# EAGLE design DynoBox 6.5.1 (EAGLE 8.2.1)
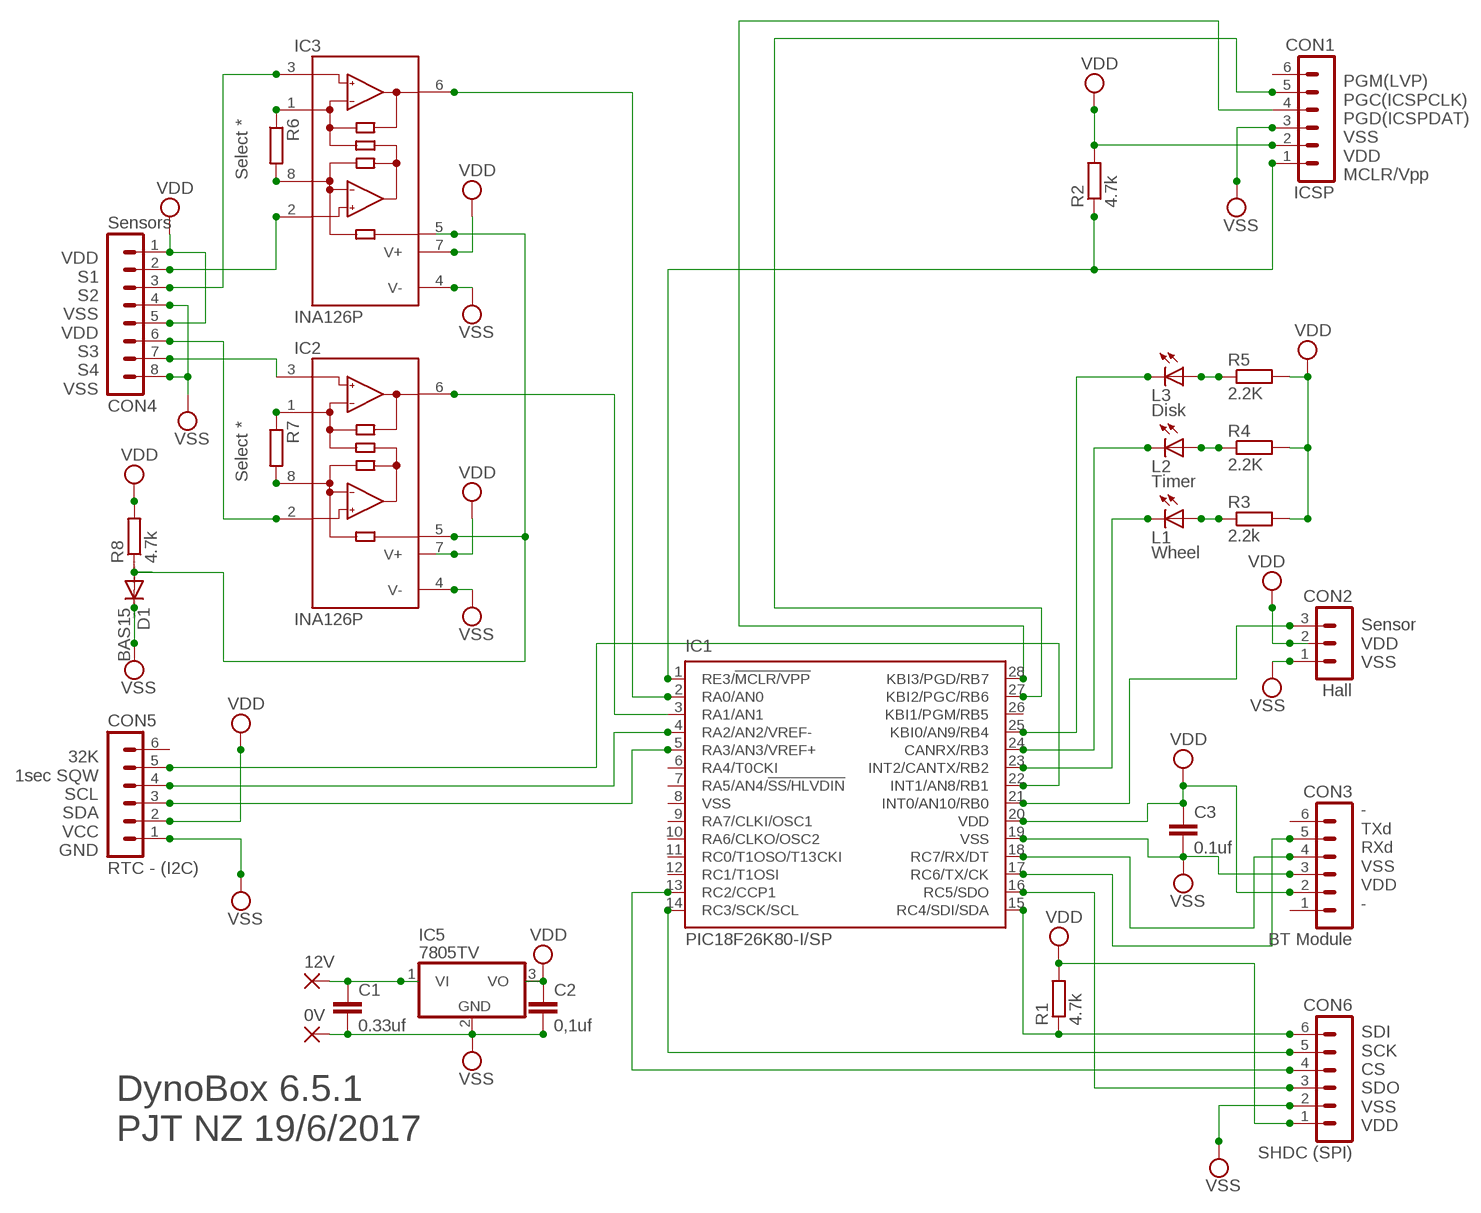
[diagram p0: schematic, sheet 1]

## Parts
0V  1,6/0,9  [1,6/0,9]
12V  1,6/0,9  [1,6/0,9]
C1  0.33uf  C-EU025-040X050  [C025-040X050]
C2  0,1uf  C-EU025-040X050  [C025-040X050]
C3  0.1uf  C-EU025-025X050  [C025-025X050]
CON1  ICSP  MA06-1  [MA06-1]
CON2  Hall  MA03-1  [MA03-1]
CON3  BT Module  MA06-1  [MA06-1]
CON4  Sensors  MA08-1  [MA08-1]
CON5  RTC - (I2C)  MA06-1  [MA06-1]
CON6  SHDC (SPI)  MA06-1  [MA06-1]
D1  BAS15  [DO34-7]
IC1  PIC18F26K80-I/SP  PIC18F2580-I/SP  [DIL28-3]
IC2  INA126P  [DIL08]
IC3  INA126P  [DIL08]
IC5  7805TV  [TO220V]
L1  Wheel  LED3MM  [LED3MM]
L2  Timer  LED3MM  [LED3MM]
L3  Disk  LED3MM  [LED3MM]
R1  4.7k  R-EU_0204/7  [0204/7]
R2  4.7k  R-EU_0204/7  [0204/7]
R3  2.2k  R-EU_0207/2V  [0207/2V]
R4  2.2K  R-EU_0207/2V  [0207/2V]
R5  2.2K  R-EU_0207/2V  [0207/2V]
R6  Select *  R-EU_0204/7  [0204/7]
R7  Select *  R-EU_0204/7  [0204/7]
R8  4.7k  R-EU_0204/7  [0204/7]

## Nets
1SEC: CON5.5 IC1.22(INT1/AN8/RB1)
N$1: IC2.8(RG) R7.2
N$2: IC2.1(RG) R7.1
N$3: L3.A R5.1
N$4: L2.A R4.1
N$6: L1.A R3.1
N$9: D1.A IC2.5(REF) IC3.5(REF) R8.1
N$10: 12V.1(P) C1.1 IC5.1(VI)
N$11: CON1.1 IC1.1(RE3/!MCLR/VPP) R2.1
N$12: CON1.4 IC1.28(KBI3/PGD/RB7)
N$13: CON1.5 IC1.27(KBI2/PGC/RB6)
N$16: CON6.6 IC1.15(RC4/SDI/SDA) R1.1
N$17: IC1.2(RA0/AN0) IC3.6(OUT)
N$18: IC1.3(RA1/AN1) IC2.6(OUT)
N$19: CON3.4 IC1.18(RC7/RX/DT)
N$20: IC3.8(RG) R6.2
N$21: CON3.5 IC1.17(RC6/TX/CK)
N$22: CON6.5 IC1.14(RC3/SCK/SCL)
N$23: IC3.1(RG) R6.1
N$28: CON6.3 IC1.16(RC5/SDO)
N$33: IC1.24(CANRX/RB3) L2.K(C)
N$34: IC1.23(INT2/CANTX/RB2) L1.K(C)
N$36: CON2.3 IC1.21(INT0/AN10/RB0)
N$37: CON5.3 IC1.5(RA3/AN3/VREF+)
N$38: CON5.4 IC1.4(RA2/AN2/VREF-)
N$39: CON6.4 IC1.13(RC2/CCP1)
N$41: IC1.25(KBI0/AN9/RB4) L3.K(C)
S1: CON4.2 IC3.2(-IN)
S2: CON4.3 IC3.3(+IN)
S3: CON4.6 IC2.2(-IN)
S4: CON4.7 IC2.3(+IN)
VDD: C2.1 C3.1 CON1.2 CON2.2 CON3.2 CON4.1 CON4.5 CON5.2 CON6.1 IC1.20(VDD) IC2.7(V+) IC3.7(V+) IC5.3(VO) R1.2 R2.2 R3.2 R4.2 R5.2 R8.2
VSS: 0V.1(P) C1.2 C2.2 C3.2 CON1.3 CON2.1 CON3.3 CON4.4 CON4.8 CON5.1 CON6.2 D1.C IC1.19(VSS) IC2.4(V-) IC3.4(V-) IC5.2(GND)
Unconnected: CON1.6 CON3.1 CON3.6 CON5.6 IC1.6(RA4/T0CKI) IC1.7(RA5/AN4/!SS/HLVDIN) IC1.9(RA7/CLKI/OSC1) IC1.10(RA6/CLKO/OSC2) IC1.11(RC0/T1OSO/T13CKI) IC1.12(RC1/T1OSI) IC1.26(KBI1/PGM/RB5)

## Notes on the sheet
- PGM(LVP)
  PGC(ICSPCLK)
  PGD(ICSPDAT)
  VSS
  VDD
  MCLR/Vpp
- VDD
  S1
  S2
  VSS
  VDD
  S3
  S4
  VSS
- Sensor
  VDD
  VSS
- 32K
  1sec SQW
  SCL
  SDA
  VCC
  GND
- -
  TXd
  RXd
  VSS
  VDD
  -
- SDI
  SCK
  CS
  SDO
  VSS
  VDD
- DynoBox 6.5.1
  PJT NZ 19/6/2017

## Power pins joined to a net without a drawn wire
VSS: IC1.8(VSS)

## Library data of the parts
0V 12V = wirepad:1,6/0,9: THROUGH-HOLE PAD
C1 C2 = rcl:C-EU: CAPACITOR, European symbol
C3 = resistor:C-EU: CAPACITOR, European symbol
CON1 CON3 CON5 CON6 = con-lstb:MA06-1: PIN HEADER; OC_FARNELL: unknown; OC_NEWARK: unknown
CON2 = con-lstb:MA03-1: PIN HEADER; OC_FARNELL: unknown; OC_NEWARK: unknown
CON4 = con-lstb:MA08-1: PIN HEADER; OC_FARNELL: unknown; OC_NEWARK: unknown
D1 = diode:BAS15: DIODE
IC1 = microchip:PIC18F2*80: 28-Pin Enhanced Flash Microcontrollers with ECAN(TM) Technology 10-Bit A/D and nanoWatt Technology Source: http://www.microchip.com .. 39637a.pdf; MF: MICROCHIP; MPN: PIC18F2580-I/SP; OC_FARNELL: 9321276; OC_NEWARK: 71J7244
IC2 IC3 = __Petes:INA126: Instrumentation Amplifier Micropower, Single and Dual Versions; MF: TEXAS INSTRUMENT CONNECTORS; MPN: INA126P; OC_FARNELL: 1509595; OC_NEWARK: 74C9780
IC5 = linear:78*: Positive VOLTAGE REGULATOR Source: http://cache.national.com/ds/LM/LM78L05.pdf http://www.fairchildsemi.com/ds/LM/LM7805.pdf
L1-L3 = led:LED: LED
R1-R8 = resistor:R-EU_: RESISTOR, European symbol

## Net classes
0 default: clearance 0.205 mm

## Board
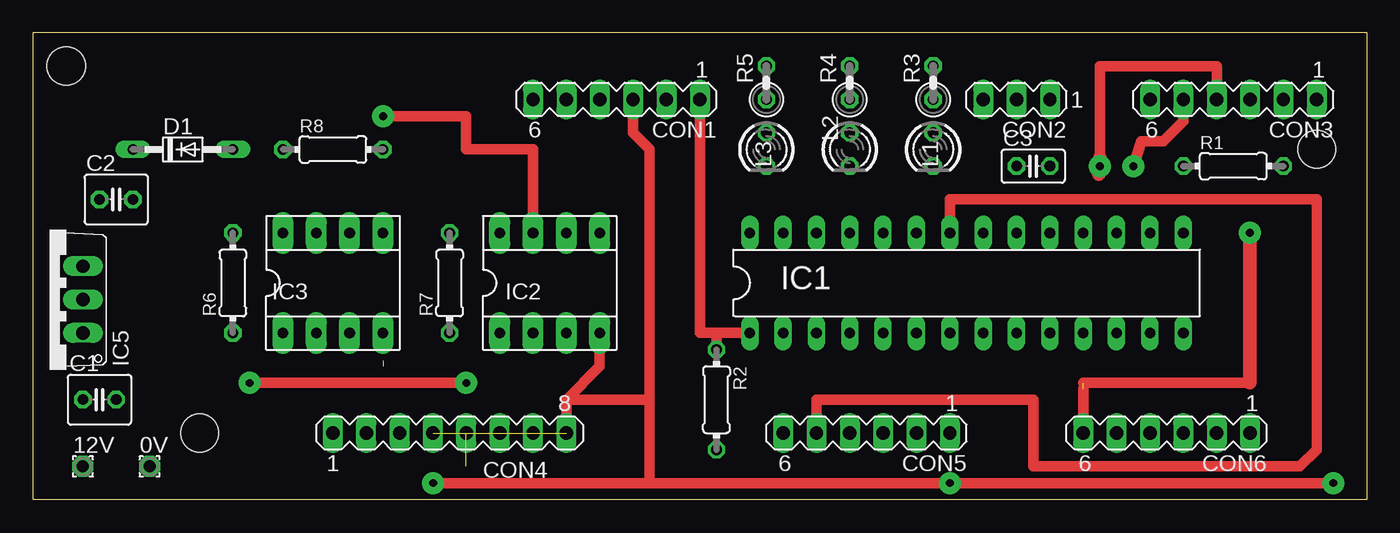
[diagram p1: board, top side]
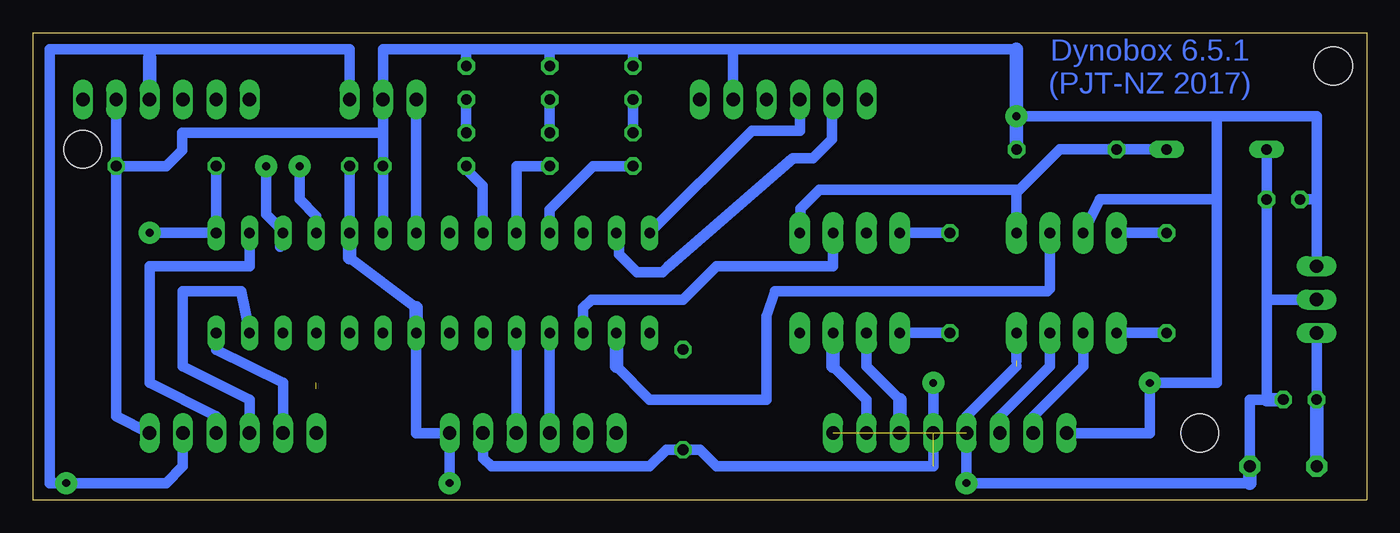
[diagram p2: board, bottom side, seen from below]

Size 101.6 x 35.56 mm. Coordinates in mm from the lower left corner, seen from the top.
Outline: 0,0.01 0,35.56 101.6,35.56 101.6,0.01
Outline: 101.6,0 0,0
Copper layers (1*16): Top 0.035mm / dielectric 1.5mm / Bottom 0.035mm
Design rules "default *": minimum track width 40mil, minimum drill 24mil, track to track 50mil, track to pad 50mil, pad to pad 50mil, via to via 50mil, smd to smd 8mil, copper to edge 40mil, drill to drill 8mil, minimum pad ring 10mil, minimum via ring 8mil, stop-mask expansion 4mil, vias tented up to drill 0mil, thermal gap 20mil
Holes 2.87 mm at 12.7,5.09 97.79,26.68
Holes 2.92 mm at 2.54,33.03

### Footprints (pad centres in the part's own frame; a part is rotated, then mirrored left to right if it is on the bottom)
1,6/0,9 = drill 0.914 pad 1.6 octagon: 1 0,0
C025-040X050 = drill 0.813 octagon: 1 -1.27,0; 2 1.27,0
C025-025X050 = drill 0.813 octagon: 1 -1.27,0; 2 1.27,0
MA06-1 = drill 1.016 long: 1 -6.35,0; 2 -3.81,0; 3 -1.27,0; 4 1.27,0; 5 3.81,0; 6 6.35,0
MA03-1 = drill 1.016 long: 1 -2.54,0; 2 0,0; 3 2.54,0
MA08-1 = drill 1.016 long: 1 -8.89,0; 2 -6.35,0; 3 -3.81,0; 4 -1.27,0; 5 1.27,0; 6 3.81,0; 7 6.35,0; 8 8.89,0
DO34-7 = drill 0.813 long: A 3.81,0; C -3.81,0
DIL28-3 = drill 0.813 long: 1 -16.51,-3.81; 2 -13.97,-3.81; 3 -11.43,-3.81; 4 -8.89,-3.81; 5 -6.35,-3.81; 6 -3.81,-3.81; 7 -1.27,-3.81; 8 1.27,-3.81; 9 3.81,-3.81; 10 6.35,-3.81; 11 8.89,-3.81; 12 11.43,-3.81; 13 13.97,-3.81; 14 16.51,-3.81; 15 16.51,3.81; 16 13.97,3.81; 17 11.43,3.81; 18 8.89,3.81; 19 6.35,3.81; 20 3.81,3.81; 21 1.27,3.81; 22 -1.27,3.81; 23 -3.81,3.81; 24 -6.35,3.81; 25 -8.89,3.81; 26 -11.43,3.81; 27 -13.97,3.81; 28 -16.51,3.81
DIL08 = drill 0.813 pad 1.6 long: 1 -3.81,-3.81; 2 -1.27,-3.81; 3 1.27,-3.81; 4 3.81,-3.81; 5 3.81,3.81; 6 1.27,3.81; 7 -1.27,3.81; 8 -3.81,3.81
TO220V = drill 1.016 long: 1 -2.54,-2.54; 2 0,-2.54; 3 2.54,-2.54
LED3MM = drill 0.813 octagon: A -1.27,0; K 1.27,0
0204/7 = drill 0.813 octagon: 1 -3.81,0; 2 3.81,0
0207/2V = drill 0.813 octagon: 1 -1.27,0; 2 1.27,0

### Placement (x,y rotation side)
0V  8.89,2.55 0 top
12V  3.81,2.55 0 top
C1  5.08,7.63 0 top
C2  6.35,22.87 0 top
C3  76.2,25.41 0 top
CON1  44.45,30.49 180 top
CON2  74.93,30.49 180 top
CON3  91.44,30.49 180 top
CON4  31.75,5.09 0 top
CON5  63.5,5.09 180 top
CON6  86.36,5.09 180 top
D1  11.43,26.68 0 top
IC1  71.12,16.52 0 top
IC2  39.37,16.52 0 top
IC3  22.86,16.52 0 top
IC5  1.27,15.25 90 top
L1  68.58,26.68 270 top
L2  62.23,26.68 270 top
L3  55.88,26.68 270 top
R1  91.44,25.41 0 top
R2  52.07,7.63 270 top
R3  68.58,31.76 90 top
R4  62.23,31.76 90 top
R5  55.88,31.76 90 top
R6  15.24,16.52 90 top
R7  31.75,16.52 90 top
R8  22.86,26.68 0 top

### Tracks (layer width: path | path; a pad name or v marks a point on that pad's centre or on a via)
1SEC
  Top 0.813: CON5.5 59.69,7.63 76.2,7.63 76.2,2.55 96.52,2.55 97.79,3.82 97.79,22.87 69.85,22.87 IC1.22
N$1
  Bottom 0.813: R7.2 IC2.8
N$2
  Bottom 0.813: R7.1 IC2.1
N$3
  Bottom 0.813: R5.1 L3.A
N$4
  Bottom 0.813: R4.1 L2.A
N$6
  Bottom 0.813: R3.1 L1.A
N$9
  Bottom 0.813: D1.A R8.1 23.36,26.68 26.44,23.61 | IC2.5 43.12,20.39 43.12,22.16 41.67,23.61 26.44,23.61 | IC3.5 26.67,23.38 26.44,23.61
N$10
  Bottom 0.813: IC5.1 C1.1 3.81,3.82
  Bottom 1.016: C1.1 12V.1
N$11
  Top 0.813: CON1.1 50.8,12.71 52.07,12.71 | 52.07,12.71 IC1.1 | R2.1 52.07,12.71
N$12
  Bottom 0.813: CON1.4 43.18,28.1 46.84,28.1 IC1.28
N$13
  Bottom 0.813: CON1.5 40.74,30.39 40.74,27.45 42.17,26.02 43.69,26.02 53.26,17.71 53.64,17.33 55.58,17.33 56.95,18.7 56.95,20.13 IC1.27
N$16  (via drill 0.6 pad 1.68)  (1 unrouted)
  Top 0.813: 80.01,8.9 92.71,8.9 | CON6.6 80.01,8.44
  Top 1.016: 92.71,8.9 v92.71,20.33
  Bottom 0.813: R1.1 IC1.15 v92.71,20.33
N$17
  Bottom 0.813: 57.15,10.17 54.61,7.63 45.72,7.63 45.72,13.98 45.09,15.88 24.33,15.88 24.13,16.09 IC3.6
  Bottom 1.016: IC1.2 57.15,10.17
N$18
  Bottom 0.813: IC2.6 40.64,17.79 49.53,17.79 52.07,15.25 59.05,15.25 59.69,14.62 IC1.3
N$19  (via drill 0.6 pad 1.68)
  Top 0.813: 81.28,26.05 81.28,33.03 90.17,33.03 CON3.4 | v81.28,25.41 81.28,25.3
  Top 1.016: v81.28,25.41 81.28,26.05 | 81.28,25.3 81.2,25.22 81.2,24.78
  Bottom 0.813: v81.28,25.41 81.28,22.87 80.01,21.6 IC1.18
N$20
  Bottom 0.813: R6.2 IC3.8
N$21  (via drill 0.6 pad 1.68)
  Top 0.813: CON3.5 87.63,28.82 86.1,27.29 84.43,27.29 v83.82,25.41
  Bottom 0.813: v83.82,25.41 83.82,21.76 82.75,20.69 82.75,19.26 IC1.17
N$22
  Bottom 0.813: CON6.5 82.55,8.9 87.63,11.44 IC1.14
N$23
  Bottom 0.813: R6.1 IC3.1
N$28
  Bottom 0.813: IC1.16 85.09,17.79 92.71,17.79 92.71,8.9 87.63,6.36 CON6.3
N$33
  Bottom 0.813: 64.57,20.53 IC1.24 64.77,25.41 L2.K
N$34
  Bottom 0.813: L1.K 68.58,25.16 67.33,23.91 67.33,20.36 IC1.23
N$36
  Bottom 0.813: CON2.3 IC1.21
N$37
  Bottom 0.813: CON5.3 IC1.5
N$38
  Bottom 0.813: CON5.4 IC1.4
N$39
  Bottom 0.813: CON6.4 85.09,7.63 90.17,10.17 90.17,15.88 85.72,15.88 IC1.13
N$41
  Bottom 0.813: L3.K 58.92,25.41 62.23,22.11 IC1.25
S1
  Bottom 0.813: CON4.2 25.4,6.36 21.59,10.17 IC3.2
S2
  Bottom 0.813: IC3.3 24.13,10.17 27.94,6.36 CON4.3
S3
  Bottom 0.813: 35.56,7.63 38.1,10.17 IC2.2
  Bottom 1.016: CON4.6 35.56,7.63
S4
  Bottom 0.813: CON4.7 38.1,7.63 40.64,10.17
  Bottom 1.016: 40.64,10.17 IC2.3
VDD  (via drill 0.6 pad 1.68)  (1 unrouted)
  Top 0.813: v16.51,8.9 v33.02,8.9 | v26.67,29.22 33.02,29.22 33.02,26.68 38.1,26.68 IC2.7
  Bottom 0.813: CON5.2 67.31,3.18 66.67,2.55 54.61,2.55 53.34,3.82 R2.2 50.8,3.82 49.53,2.55 33.02,2.55 v33.02,8.9 | CON1.2 48.26,34.3 | 48.26,34.3 26.67,34.3 | R1.2 95.25,6.36 CON6.1 | IC1.20 C3.1 74.93,27.95 | 74.93,27.95 CON2.2 74.93,34.3 68.58,34.3 | R1.2 CON3.2 | 3.81,22.87 3.81,29.22 11.43,29.22 | 11.43,29.22 11.43,22.87 | 11.43,22.87 11.43,8.9 v16.51,8.9 16.51,5.09 CON4.1 | 11.43,22.87 20.32,22.87 IC3.7 | 11.43,29.22 v26.67,29.22 | IC5.3 3.81,22.87 | 3.81,22.87 C2.1 | 48.26,34.3 55.88,34.3 | R5.2 55.88,34.3 | 55.88,34.3 62.23,34.3 | R4.2 62.23,34.3 | 62.23,34.3 68.58,34.3 | R3.2 68.58,34.3 | R1.2 91.44,25.41 90.22,26.62 90.22,27.95 74.93,27.95
  Bottom 1.016: 26.67,34.3 v26.67,29.22 R8.2
VSS  (via drill 0.6 pad 1.68)  (2 unrouted)
  Top 0.813: 46.99,7.63 46.99,1.42 | 46.99,7.63 46.99,26.68 45.72,27.95 CON1.3 | v99.06,1.28 v69.85,1.28 v30.48,1.28 | IC2.4 43.18,10.17 40.64,7.63 | 40.64,7.63 CON4.8 | 40.64,7.63 46.99,7.63
  Bottom 0.813: C3.2 IC1.19 | 77.47,18.43 72.39,14.62 72.39,5.09 CON5.1 v69.85,1.28 | 8.89,1.28 v30.48,1.28 CON4.4 30.48,6.36 26.67,10.17 | D1.C C2.2 7.62,15.25 | 0V.1 8.89,7.63 7.62,7.63 7.62,15.25 | IC5.2 7.62,15.25 | CON3.3 92.71,34.3 | 92.71,34.3 100.33,34.3 100.33,1.28 v99.06,1.28 91.44,1.28 90.17,2.55 CON6.2 | 92.71,34.3 77.47,34.3 CON2.1 | IC3.4 26.67,10.58
  Bottom 1.016: 77.47,18.43 IC1.19 | IC1.8 72.39,14.62 | 8.89,1.28 0V.1 | 92.71,33.66 CON3.3 | 7.62,7.63 C1.2

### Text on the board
Bottom: Dynobox 6.5.1 / (PJT-NZ 2017)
